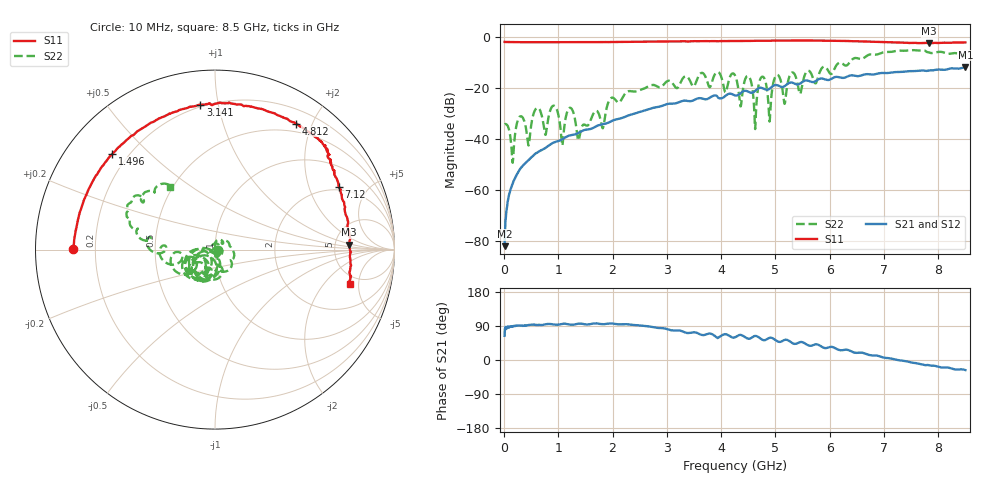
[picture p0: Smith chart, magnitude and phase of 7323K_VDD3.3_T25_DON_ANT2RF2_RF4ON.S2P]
!Agilent Technologies,E5071C,MY46417908,A.11.23
!Date: Mon Jan 18 17:06:33 2021
!Data & Calibration Information:
!Freq	S11:SOLT2(ON)	S21:SOLT2(ON)	S12:SOLT2(ON)	S22:SOLT2(ON)
!PortZ  Port1:50+j0  Port2:50+j0
!Above PortZ is port z conversion or system Z0 setting when saving the data.
!When reading, reference impedance value at option line is always used.
# Hz S dB R 50
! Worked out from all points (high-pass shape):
!   1601 points, 10 MHz to 8.5 GHz, reference 50 ohm
!   highest |S21| = -11.82 dB at 8.5 GHz (marker M1); lowest = -82.1 dB at 10 MHz (marker M2)
!   |S21| within 3 dB of the highest: 6.635 GHz to 6.779 GHz (144.3 MHz wide, 2.15 % of centre); 6.783 GHz to end of sweep
!   lowest |S11| = -2.5 dB at 7.831 GHz (marker M3), VSWR 6.94, Z = 341 + j43.6 ohm
!   |S11| at or under -10 dB: nowhere
!   |S22| runs from -49.4 to -5.2 dB; largest |S21 - S12| = 0.0036
!   S11 on the Smith chart (normalised r, x): 10 MHz: 0.12, +0.00; 1.496 GHz: 0.14, +0.39; 3.141 GHz: 0.19, +0.89; 4.812 GHz: 0.38, +1.77; 7.12 GHz: 1.83, +3.20; 8.5 GHz: 4.08, -3.88
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1e7  -2.04 179.7  -82.13 63.7  -83.31 63.3  -34.29 -2.4
1.58575e8  -2.09 175.3  -57.57 87.6  -57.66 90.0  -49.42 5.2
3.177625e8  -2.14 170.7  -51.23 91.2  -51.30 90.5  -31.16 3.9
4.451125e8  -2.14 167.2  -48.53 92.2  -48.51 91.9  -42.25 -10.4
6.096062e8  -2.16 162.6  -45.49 92.4  -45.48 92.5  -27.95 -7.7
1.426769e9  -2.13 139.1  -37.04 95.6  -37.04 95.7  -35.70 20.1
1.49575e9  -2.13 137.2  -36.52 94.2  -36.51 93.9  -34.55 -58.3
2.843538e9  -1.90 101.8  -27.49 84.5  -27.49 84.6  -19.77 -36.0
3.140688e9  -1.81 95.8  -26.19 77.8  -26.19 77.8  -19.37 -79.4
4.255e9  -1.66 70.9  -23.00 59.9  -23.01 59.9  -15.16 -162.0
4.355819e9  -1.66 68.0  -22.15 66.3  -22.17 66.2  -27.33 -147.3
4.515006e9  -1.64 64.1  -21.70 56.0  -21.71 56.0  -15.70 -151.7
4.626438e9  -1.60 61.4  -21.23 63.5  -21.25 63.3  -36.21 -130.4
4.812156e9  -1.56 57.1  -20.67 52.7  -20.68 52.5  -17.27 -152.6
4.89175e9  -1.56 55.1  -20.37 58.5  -20.38 58.4  -33.26 -122.5
5.0191e9  -1.52 53.5  -18.96 50.9  -18.96 50.9  -15.07 -110.2
5.167675e9  -1.49 49.9  -19.39 53.0  -19.39 52.8  -26.33 -122.6
5.671769e9  -1.49 43.5  -17.75 38.1  -17.72 38.0  -15.07 -162.5
7.088538e9  -2.17 27.9  -14.19 4.8  -14.24 4.6  -5.98 160.3
7.120375e9  -2.23 26.9  -14.08 4.2  -14.11 4.1  -5.97 160.2
7.831412e9  -2.52 2.2  -13.22 -13.9  -13.23 -13.7  -6.17 145.1
8.5e9  -2.22 -14.2  -11.82 -26.6  -11.92 -26.7  -7.30 125.7
